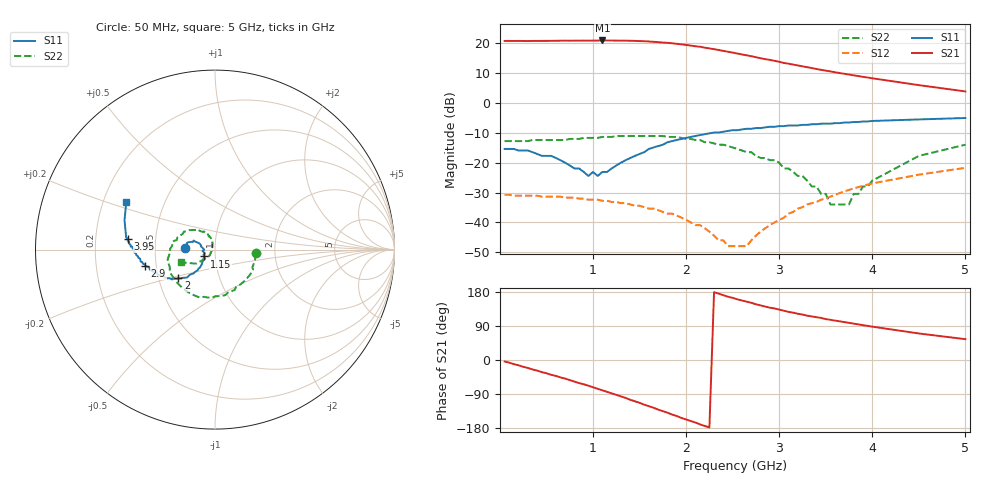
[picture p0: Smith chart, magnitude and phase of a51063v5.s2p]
!  INA-51063 S PARAMETERS
!  Vd = 5 V  LAST UPDATED 03-20-96
# ghz s ma r 50
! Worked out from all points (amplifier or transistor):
!   82 points, 50 MHz to 5 GHz, reference 50 ohm
!   highest |S21| = 20.9 dB at 1.1 GHz (marker M1)
!   |S21| within 3 dB of that: start of sweep to 2.315 GHz
!   unconditionally stable (mu >= 1): start of sweep to end of sweep
!   at 700 MHz: K = 1.79, MAG = 21.1 dB, |S12| = -31.7 dB
!   at 2.1 GHz: K = 5.49, MAG = 19.6 dB, |S12| = -40.9 dB
!   at 5 GHz: K = 2.75, MAG = 5.5 dB, |S12| = -21.7 dB
!   lowest NFmin = 2.16 dB at 600 MHz
!   S11 on the Smith chart (normalised r, x): 50 MHz: 0.71, +0.01; 1.15 GHz: 0.89, -0.07; 2 GHz: 0.63, -0.22; 2.9 GHz: 0.43, -0.09; 3.95 GHz: 0.34, +0.05; 5 GHz: 0.30, +0.23
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0.05  0.17 177.0  10.94 -4.0  0.029 -1.0  0.23 -5.0
0.2  0.16 170.0  10.94 -14.0  0.028 -4.0  0.23 -16.0
0.5  0.13 159.0  10.96 -35.0  0.027 -9.0  0.24 -43.0
0.7  0.1 158.0  11.06 -49.0  0.026 -12.0  0.24 -61.0
0.9  0.07 172.0  11.1 -64.0  0.025 -15.0  0.26 -77.0
1.1  0.07 -156.0  11.14 -80.0  0.023 -18.0  0.27 -94.0
1.15  0.07 -147.0  11.13 -84.0  0.023 -20.0  0.27 -99.0
1.3  0.1 -135.0  11.08 -96.0  0.021 -23.0  0.28 -113.0
1.45  0.13 -130.0  10.95 -109.0  0.019 -27.0  0.28 -126.0
1.6  0.17 -132.0  10.71 -122.0  0.017 -30.0  0.28 -140.0
1.7  0.19 -134.0  10.45 -131.0  0.016 -33.0  0.28 -150.0
1.85  0.23 -137.0  9.99 -144.0  0.014 -37.0  0.27 -163.0
2  0.26 -142.0  9.37 -157.0  0.011 -42.0  0.25 -177.0
2.15  0.29 -145.0  8.75 -170.0  0.009 -51.0  0.24 169.0
2.25  0.31 -149.0  8.2 -178.0  0.007 -58.0  0.22 162.0
2.55  0.35 -158.0  6.73 160.0  0.004 -127.0  0.17 140.0
2.9  0.4 -167.0  5.26 138.0  0.009 167.0  0.11 119.0
3.35  0.44 -176.0  3.84 115.0  0.021 148.0  0.04 109.0
3.55  0.45 -180.0  3.37 106.0  0.027 145.0  0.02 133.0
3.95  0.49 173.0  2.67 90.0  0.043 133.0  0.04 -134.0
4.5  0.53 162.0  1.99 70.0  0.063 118.0  0.13 -143.0
5  0.56 152.0  1.56 55.0  0.082 108.0  0.2 -159.0
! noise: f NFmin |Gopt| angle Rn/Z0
0.6  2.16  0.19  44  0.33
0.9  2.26  0.25  63  0.32
1.8  2.89  0.28  120  0.27
2.4  3.45  0.34  152  0.24
